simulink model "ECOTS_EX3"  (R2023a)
settings: Solver=ode23tb  StartTime=0.0  StopTime=meas.Time(end)  RelTol=1e-3
undefined symbols (not defined in the file or in its folder): mm
libraries: component_lib x10

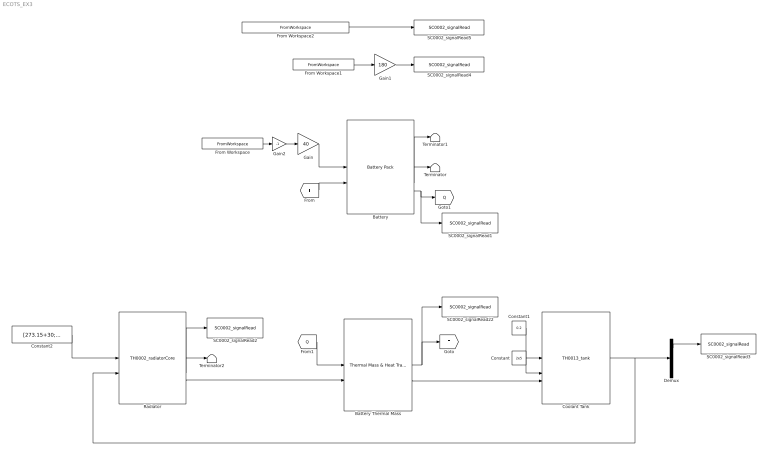
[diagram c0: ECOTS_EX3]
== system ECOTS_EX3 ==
  Battery : component_lib/Battery Pack  SOC_0=1  Nx=40  Ny=180
  Battery Thermal Mass : component_lib/Thermal Mass & Heat Transfer  n=100  d=10e-3  L=4  m=40 * 180 * 0.048  cp=1040  T_0=273 + 25
  Constant : Constant  Value=2e5
  Constant1 : Constant  Value=0.2
  Constant2 : Constant  Value=[273.15+30; 1e5; 5]
  Coolant Tank : component_lib/Thermal Systems/TH0013_tank  V=5e-3  T0=273.15 + 25
  Demux : Demux  Outputs=3
  From Workspace : FromWorkspace  VariableName=[meas.Time, meas.Current]
  From Workspace1 : FromWorkspace  VariableName=[meas.Time, meas.Voltage]
  From Workspace2 : FromWorkspace  VariableName=[meas.Time, meas.Battery_Temp_degC + 273.15]
  Gain : Gain  Gain=40
  Gain1 : Gain  Gain=180
  Gain2 : Gain  Gain=-1
  Radiator : component_lib/Thermal Systems/TH0002_radiatorCore  HtH=1.1  StS=0.95  radmodel=52 mm
  SC0002_signalRead1 : component_lib/Data & Control/SC0002_signalRead  SigName=generatedHeat
  SC0002_signalRead2 : component_lib/Data & Control/SC0002_signalRead  SigName=radiatorCooling
  SC0002_signalRead22 : component_lib/Data & Control/SC0002_signalRead  SigName=batteryTemperature
  SC0002_signalRead3 : component_lib/Data & Control/SC0002_signalRead  SigName=coolantTemperature
  SC0002_signalRead4 : component_lib/Data & Control/SC0002_signalRead  SigName=measuredBatteryVoltage
  SC0002_signalRead5 : component_lib/Data & Control/SC0002_signalRead  SigName=measuredBatteryTemperature
  Terminator : Terminator
  Terminator1 : Terminator
  Terminator2 : Terminator
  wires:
  Battery/2 -> Terminator/1
  Battery/1 -> Terminator1/1
  Battery Thermal Mass/2 -> Coolant Tank/3
  Battery Thermal Mass/1 -> [T], SC0002_signalRead22/1
  [T] -> Battery/2
  Battery/3 -> SC0002_signalRead1/1, [Q]
  [Q] -> Battery Thermal Mass/1
  Constant/1 -> Coolant Tank/2
  Constant1/1 -> Coolant Tank/1
  Radiator/3 -> Battery Thermal Mass/2
  Coolant Tank/1 -> Demux/1, Radiator/2
  Constant2/1 -> Radiator/1
  Radiator/2 -> Terminator2/1
  Radiator/1 -> SC0002_signalRead2/1
  Demux/1 -> SC0002_signalRead3/1
  Gain1/1 -> SC0002_signalRead4/1
  From Workspace2/1 -> SC0002_signalRead5/1
  From Workspace1/1 -> Gain1/1
  Gain2/1 -> Gain/1
  From Workspace/1 -> Gain2/1
  Gain/1 -> Battery/1
